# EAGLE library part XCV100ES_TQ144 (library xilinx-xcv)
xcv100es_tq144 edit this description Auto generated by make-symbol-device-package-bsdl.ulp Rev. 26 Source: xcv100es_tq144.bsd
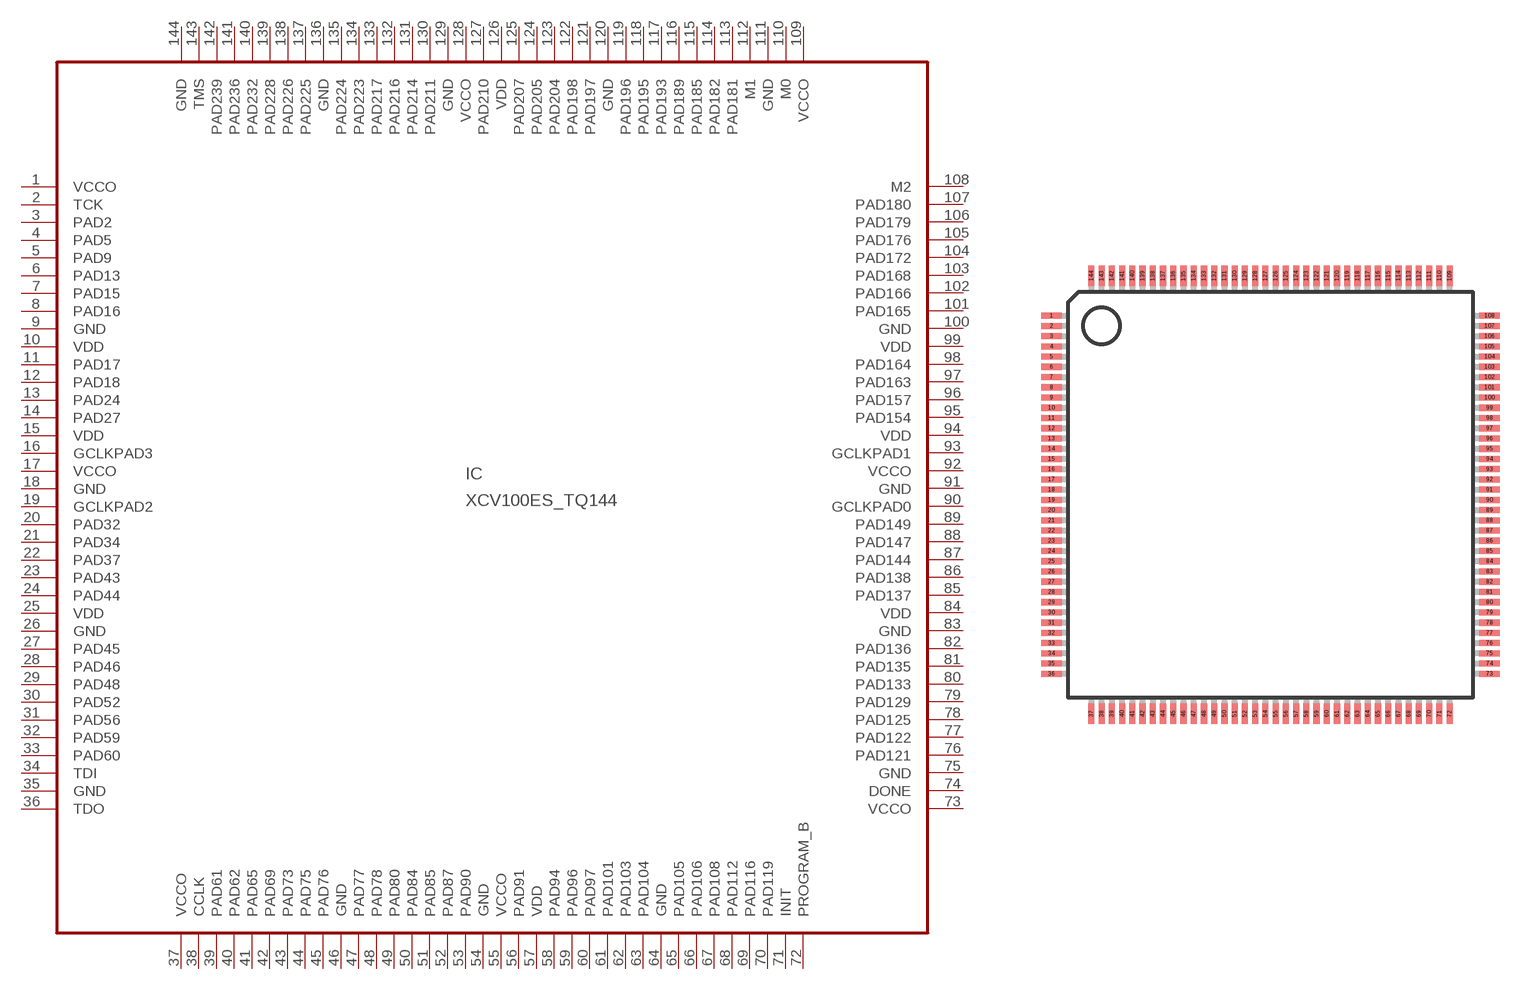
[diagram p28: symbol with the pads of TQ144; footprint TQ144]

Designator prefix IC

## XCV100ES_TQ144 (OC_FARNELL: unknown; OC_NEWARK: unknown)  [TQ144]
1  VCCO  pwr
2  TCK  in
3  PAD2
4  PAD5
5  PAD9
6  PAD13
7  PAD15
8  PAD16
9  GND  pwr
10  VDD  pwr
11  PAD17
12  PAD18
13  PAD24
14  PAD27
15  VDD  pwr
16  GCLKPAD3  in
17  VCCO  pwr
18  GND  pwr
19  GCLKPAD2  in
20  PAD32
21  PAD34
22  PAD37
23  PAD43
24  PAD44
25  VDD  pwr
26  GND  pwr
27  PAD45
28  PAD46
29  PAD48
30  PAD52
31  PAD56
32  PAD59
33  PAD60
34  TDI  in
35  GND  pwr
36  TDO  out
37  VCCO  pwr
38  CCLK
39  PAD61
40  PAD62
41  PAD65
42  PAD69
43  PAD73
44  PAD75
45  PAD76
46  GND  pwr
47  PAD77
48  PAD78
49  PAD80
50  PAD84
51  PAD85
52  PAD87
53  PAD90
54  GND  pwr
55  VCCO  pwr
56  PAD91
57  VDD  pwr
58  PAD94
59  PAD96
60  PAD97
61  PAD101
62  PAD103
63  PAD104
64  GND  pwr
65  PAD105
66  PAD106
67  PAD108
68  PAD112
69  PAD116
70  PAD119
71  INIT
72  PROGRAM_B  in
73  VCCO  pwr
74  DONE
75  GND  pwr
76  PAD121
77  PAD122
78  PAD125
79  PAD129
80  PAD133
81  PAD135
82  PAD136
83  GND  pwr
84  VDD  pwr
85  PAD137
86  PAD138
87  PAD144
88  PAD147
89  PAD149
90  GCLKPAD0  in
91  GND  pwr
92  VCCO  pwr
93  GCLKPAD1  in
94  VDD  pwr
95  PAD154
96  PAD157
97  PAD163
98  PAD164
99  VDD  pwr
100  GND  pwr
101  PAD165
102  PAD166
103  PAD168
104  PAD172
105  PAD176
106  PAD179
107  PAD180
108  M2  in
109  VCCO  pwr
110  M0  in
111  GND  pwr
112  M1  in
113  PAD181
114  PAD182
115  PAD185
116  PAD189
117  PAD193
118  PAD195
119  PAD196
120  GND  pwr
121  PAD197
122  PAD198
123  PAD204
124  PAD205
125  PAD207
126  VDD  pwr
127  PAD210
128  VCCO  pwr
129  GND  pwr
130  PAD211
131  PAD214
132  PAD216
133  PAD217
134  PAD223
135  PAD224
136  GND  pwr
137  PAD225
138  PAD226
139  PAD228
140  PAD232
141  PAD236
142  PAD239
143  TMS  in
144  GND  pwr

## Footprint TQ144 (pad centres in mm)
TQ144 Auto generated by make-symbol-device-package-bsdl.ulp Rev. 26 Source: xcv100_tq144_1532.bsd; tq144.pdf
smd 1 x 0.3: 1 -10.7,8.75; 2 -10.7,8.25; 3 -10.7,7.75; 4 -10.7,7.25; 5 -10.7,6.75; 6 -10.7,6.25; 7 -10.7,5.75; 8 -10.7,5.25; 9 -10.7,4.75; 10 -10.7,4.25; 11 -10.7,3.75; 12 -10.7,3.25; 13 -10.7,2.75; 14 -10.7,2.25; 15 -10.7,1.75; 16 -10.7,1.25; 17 -10.7,0.75; 18 -10.7,0.25; 19 -10.7,-0.25; 20 -10.7,-0.75; 21 -10.7,-1.25; 22 -10.7,-1.75; 23 -10.7,-2.25; 24 -10.7,-2.75; 25 -10.7,-3.25; 26 -10.7,-3.75; 27 -10.7,-4.25; 28 -10.7,-4.75; 29 -10.7,-5.25; 30 -10.7,-5.75; 31 -10.7,-6.25; 32 -10.7,-6.75; 33 -10.7,-7.25; 34 -10.7,-7.75; 35 -10.7,-8.25; 36 -10.7,-8.75; 73 10.7,-8.75; 74 10.7,-8.25; 75 10.7,-7.75; 76 10.7,-7.25; 77 10.7,-6.75; 78 10.7,-6.25; 79 10.7,-5.75; 80 10.7,-5.25; 81 10.7,-4.75; 82 10.7,-4.25; 83 10.7,-3.75; 84 10.7,-3.25; 85 10.7,-2.75; 86 10.7,-2.25; 87 10.7,-1.75; 88 10.7,-1.25; 89 10.7,-0.75; 90 10.7,-0.25; 91 10.7,0.25; 92 10.7,0.75; 93 10.7,1.25; 94 10.7,1.75; 95 10.7,2.25; 96 10.7,2.75; 97 10.7,3.25; 98 10.7,3.75; 99 10.7,4.25; 100 10.7,4.75; 101 10.7,5.25; 102 10.7,5.75; 103 10.7,6.25; 104 10.7,6.75; 105 10.7,7.25; 106 10.7,7.75; 107 10.7,8.25; 108 10.7,8.75
smd 0.3 x 1: 37 -8.75,-10.7; 38 -8.25,-10.7; 39 -7.75,-10.7; 40 -7.25,-10.7; 41 -6.75,-10.7; 42 -6.25,-10.7; 43 -5.75,-10.7; 44 -5.25,-10.7; 45 -4.75,-10.7; 46 -4.25,-10.7; 47 -3.75,-10.7; 48 -3.25,-10.7; 49 -2.75,-10.7; 50 -2.25,-10.7; 51 -1.75,-10.7; 52 -1.25,-10.7; 53 -0.75,-10.7; 54 -0.25,-10.7; 55 0.25,-10.7; 56 0.75,-10.7; 57 1.25,-10.7; 58 1.75,-10.7; 59 2.25,-10.7; 60 2.75,-10.7; 61 3.25,-10.7; 62 3.75,-10.7; 63 4.25,-10.7; 64 4.75,-10.7; 65 5.25,-10.7; 66 5.75,-10.7; 67 6.25,-10.7; 68 6.75,-10.7; 69 7.25,-10.7; 70 7.75,-10.7; 71 8.25,-10.7; 72 8.75,-10.7; 109 8.75,10.7; 110 8.25,10.7; 111 7.75,10.7; 112 7.25,10.7; 113 6.75,10.7; 114 6.25,10.7; 115 5.75,10.7; 116 5.25,10.7; 117 4.75,10.7; 118 4.25,10.7; 119 3.75,10.7; 120 3.25,10.7; 121 2.75,10.7; 122 2.25,10.7; 123 1.75,10.7; 124 1.25,10.7; 125 0.75,10.7; 126 0.25,10.7; 127 -0.25,10.7; 128 -0.75,10.7; 129 -1.25,10.7; 130 -1.75,10.7; 131 -2.25,10.7; 132 -2.75,10.7; 133 -3.25,10.7; 134 -3.75,10.7; 135 -4.25,10.7; 136 -4.75,10.7; 137 -5.25,10.7; 138 -5.75,10.7; 139 -6.25,10.7; 140 -6.75,10.7; 141 -7.25,10.7; 142 -7.75,10.7; 143 -8.25,10.7; 144 -8.75,10.7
